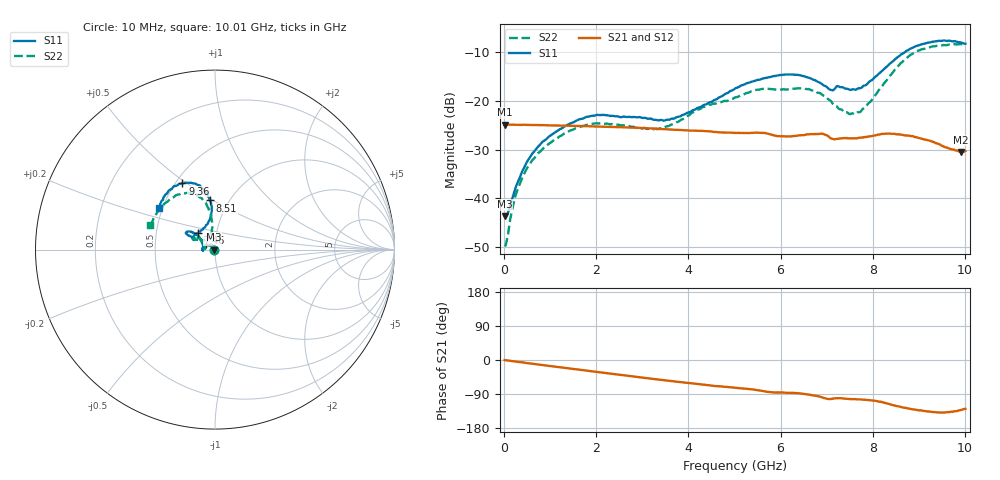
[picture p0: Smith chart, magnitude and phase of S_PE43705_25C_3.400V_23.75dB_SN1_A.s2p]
! Device ID: PE43705
! Serial: 1
! Insertion: A
! Impedance: 50 ohm
! Temp: 25C
! VDD: 3.400V
! Attenuation Step: 23.75dB
#  Hz  S  RI  R  50
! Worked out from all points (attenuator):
!   401 points, 10 MHz to 10.01 GHz, reference 50 ohm
!   highest |S21| = -24.82 dB at 10 MHz (marker M1); lowest = -30.5 dB at 9.91 GHz (marker M2)
!   lowest |S11| = -43.7 dB at 10 MHz (marker M3), VSWR 1.01, Z = 49.4 + j0.0444 ohm
!   |S11| at or under -10 dB: start of sweep to 8.683 GHz
!   |S22| runs from -49.8 to -8.3 dB; largest |S21 - S12| = 0.00072
!   S11 on the Smith chart (normalised r, x): 10 MHz: 0.99, +0.00; 7.46 GHz: 0.81, +0.16; 8.51 GHz: 0.82, +0.48; 9.36 GHz: 0.54, +0.48; 10.01 GHz: 0.48, +0.26
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1e7  -0.00653 0.00045  0.0574 -0.000223  0.0575 -0.00019  -0.00319 0.000533
8.5e7  -0.00625 0.00349  0.0573 -0.00148  0.0572 -0.00142  -0.00259 0.00339
2.6e8  -0.00778 0.0109  0.0569 -0.00427  0.0569 -0.00426  -0.00393 0.0105
5.35e8  -0.0147 0.0207  0.0562 -0.00859  0.0562 -0.0086  -0.00994 0.0192
1.01e9  -0.0356 0.0265  0.054 -0.0157  0.0542 -0.0157  -0.0281 0.0246
1.685e9  -0.0638 0.0161  0.0496 -0.0246  0.0496 -0.0246  -0.0525 0.0169
2.16e9  -0.0721 0.00245  0.0454 -0.0303  0.0455 -0.0303  -0.0581 0.00726
3.36e9  -0.0634 0.00267  0.032 -0.0407  0.0321 -0.0407  -0.0501 0.0132
3.86e9  -0.0669 0.0253  0.026 -0.0431  0.0261 -0.0429  -0.0586 0.0281
5.01e9  -0.104 0.0853  0.0136 -0.0452  0.0138 -0.0452  -0.0886 0.0635
5.535e9  -0.1334 0.0983  0.00803 -0.0464  0.00797 -0.0466  -0.1081 0.0742
6.01e9  -0.1567 0.0996  0.00328 -0.0433  0.00345 -0.0432  -0.1106 0.0712
6.685e9  -0.1481 0.0786  -0.00246 -0.0457  -0.00235 -0.0458  -0.1145 0.0583
7.085e9  -0.1154 0.0612  -0.00926 -0.0405  -0.00943 -0.0408  -0.0845 0.0549
7.46e9  -0.0943 0.0944  -0.00913 -0.0404  -0.00906 -0.0405  -0.0502 0.0567
7.785e9  -0.0514 0.1321  -0.0106 -0.0407  -0.0104 -0.041  -0.0282 0.0785
8.36e9  -0.0181 0.2393  -0.0207 -0.0416  -0.0207 -0.0415  -0.0209 0.178
8.51e9  -0.0272 0.2736  -0.0237 -0.0389  -0.0234 -0.0394  -0.0316 0.2138
8.91e9  -0.0811 0.3534  -0.028 -0.0322  -0.0278 -0.0325  -0.0981 0.3017
9.36e9  -0.1812 0.3684  -0.0274 -0.025  -0.0277 -0.0252  -0.2004 0.3073
9.91e9  -0.3007 0.2646  -0.0201 -0.0223  -0.0205 -0.0224  -0.3426 0.1772
1.001e10  -0.3138 0.2299  -0.0193 -0.0239  -0.0189 -0.0237  -0.3609 0.1373
